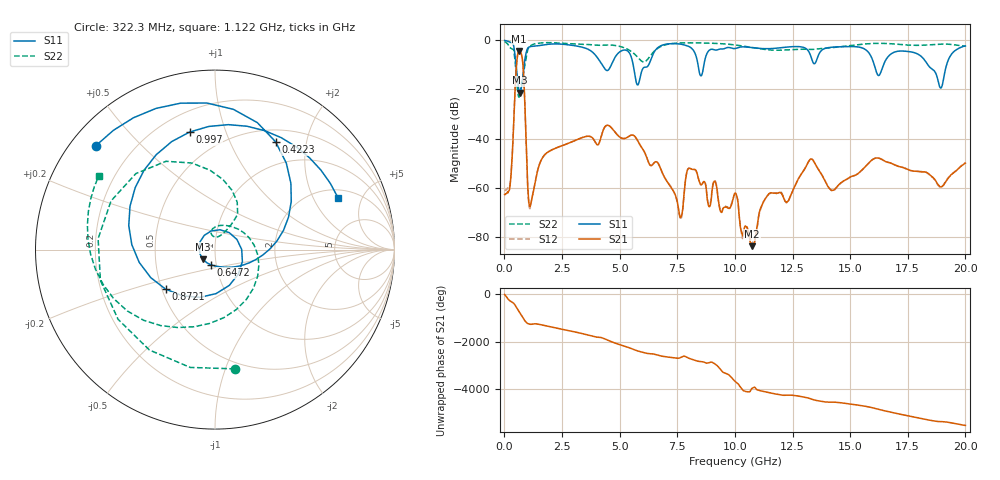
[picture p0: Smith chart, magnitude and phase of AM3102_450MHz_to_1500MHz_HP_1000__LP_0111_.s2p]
!Agilent Technologies,E8364B,MY43040894,A.07.50.67
!Agilent E8364B: A.07.50.67
!Date: Thursday, January 11, 2018 05:58:05
!Correction: S11(Full 2 Port(1,2))
!S21(Full 2 Port(1,2))
!S12(Full 2 Port(1,2))
!S22(Full 2 Port(1,2))
!S2P File: Measurements: S11, S21, S12, S22:
# Hz S  dB  R 50
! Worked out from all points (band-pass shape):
!   1601 points, 10 MHz to 20 GHz, reference 50 ohm
!   highest |S21| = -4.39 dB at 647.2 MHz (marker M1); lowest = -83.9 dB at 10.74 GHz (marker M2)
!   |S21| within 3 dB of the highest: 554 MHz to 776.1 MHz (222.2 MHz wide, 33.4 % of centre)
!   lowest |S11| = -21.3 dB at 672.2 MHz (marker M3), VSWR 1.19, Z = 43.5 - j4.66 ohm
!   |S11| at or under -10 dB: 4.244 GHz to 4.639 GHz (394.4 MHz wide, 8.88 % of centre); 5.588 GHz to 6.26 GHz (671.9 MHz wide, 11.3 % of centre); 18.37 GHz to 19.18 GHz (811.2 MHz wide, 4.32 % of centre)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
!   |S22| runs from -23.2 to -0.5 dB; largest |S21 - S12| = 0.0015
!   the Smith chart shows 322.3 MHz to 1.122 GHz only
!   S11 on the Smith chart (normalised r, x): 322.3 MHz: 0.07, +0.37; 422.3 MHz: 0.66, +1.50; 647.2 MHz: 0.94, -0.16; 872.1 MHz: 0.52, -0.26; 997 MHz: 0.32, +0.76; 1.122 GHz: 2.45, +3.17
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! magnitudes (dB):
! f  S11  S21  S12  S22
! 10 MHz  -0.1  -62.8  -61.3  -0.5
! 322.3 MHz  -1.1  -49.9  -49.8  -3.4
! 422.3 MHz  -3.2  -28.7  -28.7  -5.0
! 647.2 MHz  -21.1  -4.4  -4.4  -22.9
! 672.2 MHz  -21.3  -4.5  -4.5  -22.2
! 872.1 MHz  -9.1  -21.8  -21.8  -11.0
! 997 MHz  -3.5  -56.0  -56.8  -4.5
! 1.122 GHz  -2.6  -67.7  -68.3  -2.3
! 1.722 GHz  -1.8  -46.9  -47.0  -1.0
! 3.346 GHz  -2.7  -39.7  -39.7  -1.6
! 5.782 GHz  -18.2  -40.9  -40.9  -6.9
! 6.682 GHz  -2.8  -50.3  -50.3  -3.1
! 7.644 GHz  -1.6  -72.3  -72.9  -1.1
! 8.043 GHz  -2.7  -52.2  -52.1  -1.0
! 8.531 GHz  -14.5  -58.9  -58.9  -1.1
! 10.01 GHz  -3.4  -62.2  -62.5  -1.9
! 10.74 GHz  -3.0  -83.9  -82.1  -3.0
! 13.34 GHz  -7.8  -48.4  -48.4  -3.7
! 14.24 GHz  -2.8  -61.1  -61.3  -3.0
! 16.68 GHz  -6.3  -49.8  -49.8  -1.3
! 18.93 GHz  -19.4  -59.7  -59.8  -1.6
! 20 GHz  -2.3  -50.0  -49.9  -2.4
